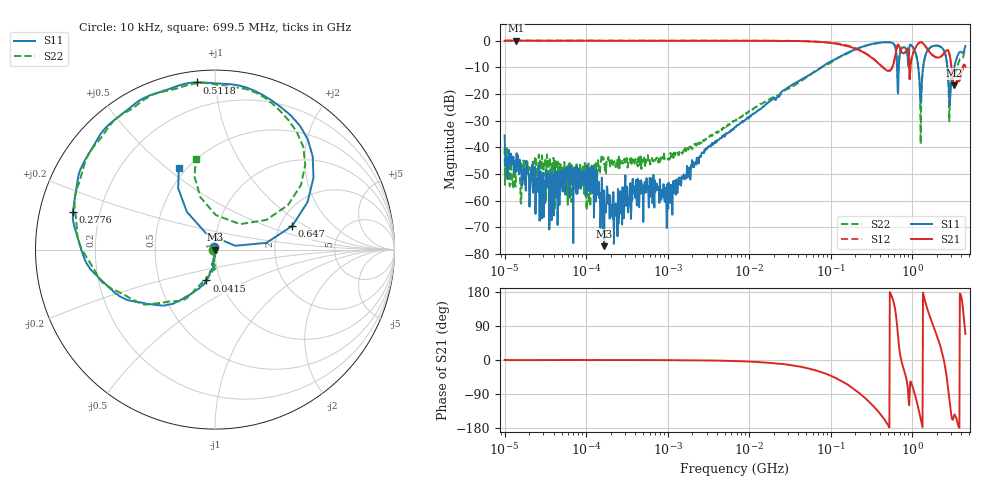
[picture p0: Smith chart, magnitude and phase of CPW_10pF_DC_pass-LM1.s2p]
!Siglent Technologies,SNA5004A,SNA5XCED5R0097,V1.0.0.2.10.R9
!Date: 2024-10-29 17:19:18
!Data & Calibration Information:
!Freq	S11:F2(ON)	S21:F2(ON)	S12:F2(ON)	S22:F2(ON)
# Hz S DB R 50
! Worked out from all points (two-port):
!   1001 points, 10 kHz to 4.5 GHz, reference 50 ohm
!   highest |S21| = -0.01 dB at 13.85 kHz (marker M1); lowest = -16.7 dB at 3.25 GHz (marker M2)
!   |S21| within 3 dB of the highest: start of sweep to 200.3 MHz; 1.085 GHz to 1.525 GHz (439.4 MHz wide, 33.7 % of centre)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
!   lowest |S11| = -77.0 dB at 166.4 kHz (marker M3), VSWR 1.00, Z = 50 + j0.00312 ohm
!   |S11| at or under -10 dB: start of sweep to 77.75 MHz; 1.189 GHz to 1.363 GHz (174.3 MHz wide, 13.7 % of centre); 2.705 GHz to 3.289 GHz (583.8 MHz wide, 19.5 % of centre)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
!   |S22| runs from -63.5 to -0.6 dB; largest |S21 - S12| = 0.032
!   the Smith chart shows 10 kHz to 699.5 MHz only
!   S11 on the Smith chart (normalised r, x): 10 kHz: 0.99, +0.03; 41.5 MHz: 0.86, -0.30; 277.6 MHz: 0.10, +0.13; 511.8 MHz: 0.06, +0.89; 647 MHz: 2.33, +0.77; 699.5 MHz: 0.45, +0.55
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10000  -35.55 110.3  -0.12 0.1  -0.04 0.3  -40.22 -166.4
13846.19  -49.18 -0.9  -0.01 -0.1  0.05 -0.2  -46.18 -30.4
37724.86  -67.31 -31.5  -0.07 -0.1  -0.01 -0.1  -47.00 -156.4
87919.76  -52.63 68.6  -0.06 0.1  -0.00 -0.0  -51.68 -170.2
166377.2  -77.05 12.8  -0.06 -0.1  -0.01 -0.1  -46.33 -150.6
772988.4  -55.87 149.9  -0.07 -0.2  -0.02 -0.3  -45.72 -147.2
6708204  -32.47 -95.9  -0.07 -2.7  -0.03 -2.8  -30.07 -101.5
4.150076e7  -14.98 -105.6  -0.19 -17.3  -0.15 -17.4  -15.60 -106.6
5.897837e7  -12.33 -113.4  -0.36 -24.7  -0.29 -24.7  -12.29 -116.3
2.776036e8  -1.74 165.2  -5.10 -104.4  -5.03 -104.3  -1.89 165.5
5.118303e8  -0.57 96.2  -11.35 -173.5  -11.25 -173.2  -0.62 97.2
5.185364e8  -0.60 94.1  -11.34 -175.8  -11.26 -175.5  -0.59 95.3
6.469696e8  -6.94 17.0  -2.63 100.1  -2.55 100.4  -6.45 31.4
6.995248e8  -6.02 113.8  -2.52 25.7  -2.43 26.1  -5.73 101.8
8.393597e8  -3.11 50.0  -4.11 -44.8  -4.02 -44.4  -3.11 45.7
1.117683e9  -5.29 -5.5  -2.29 -102.9  -2.23 -102.5  -5.34 -12.0
1.323764e9  -14.07 79.5  -0.78 -171.9  -0.72 -171.4  -14.59 95.2
1.856924e9  -1.97 -9.2  -5.92 84.4  -5.85 85.0  -1.97 -6.8
2.440684e9  -3.60 -97.7  -4.91 1.2  -4.84 2.0  -3.60 -91.0
2.779993e9  -14.42 -179.1  -3.86 -81.2  -3.78 -80.4  -16.06 -166.5
3.249991e9  -10.85 133.2  -16.72 -148.6  -16.61 -147.2  -12.29 -157.4
4.5e9  -2.03 -40.0  -9.82 68.8  -9.89 66.1  -2.49 -26.0
